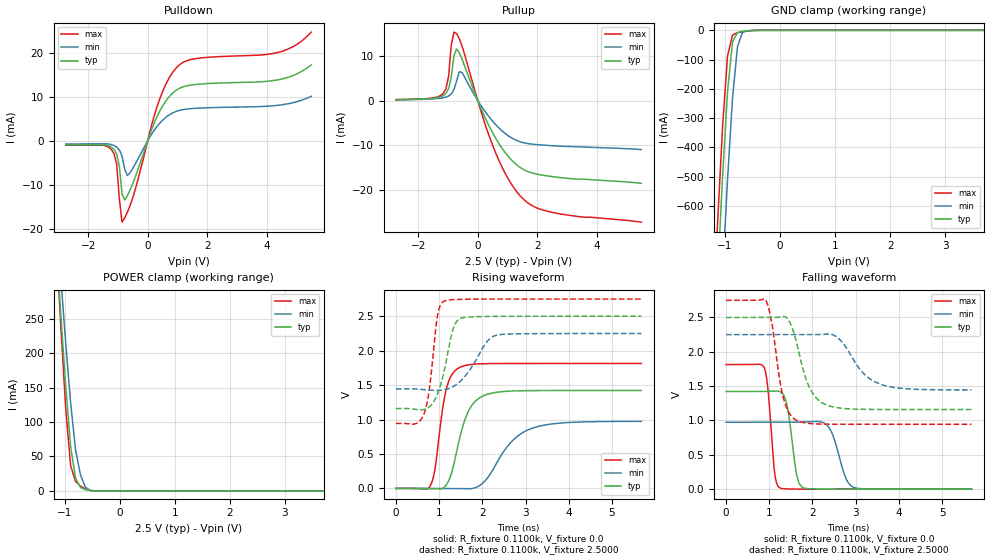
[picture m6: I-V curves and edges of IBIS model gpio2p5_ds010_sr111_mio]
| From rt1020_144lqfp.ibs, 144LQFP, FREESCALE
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[Model] gpio2p5_ds010_sr111_mio
|   Model gpio2p5_ds010_sr111_mio
| This model was characterised for following simulation conditions:
| External (pad) voltage:
|   - Typ: 2.5V,   - Min: 2.25V,   - Max: 2.75V
| Library cells for typ/min/max conditions are connected as defined below:
|  pad - External Pad
|  ipp_do - Core Input
|  ipp_obe - Output Buffer Enable
|  esd_boost - ovdd
|  ipp_dse0 - vssi
|  ipp_dse1 - vddi
|  ipp_dse2 - vssi
|  ipp_fsel0 - vddi
|  ipp_fsel1 - vddi
|  ipp_ina - ipp_ina
|  ipp_ind - ipp_ind
|  ipp_pwr_stable - vddi
|  ipp_sre - vddi
|  ovdd - ovdd
|  ovss - ovss
|  vddi - vddi
|  vssi - vssi
| All other pins connected to ground
Model_type I/O
Polarity   Non-Inverting
Enable   Active-High
Vinl =   0.7500V
Vinh =   1.7500V
Vmeas =  1.2500V
Cref =   0.0F
Rref =   0.1100k
Vref =   1.2500V
C_comp   1.2356pF   1.1994pF   1.2834pF
|C_comp_pullup   0.6222pF   0.6389pF   0.6073pF
|C_comp_pulldown   0.5474pF   0.5788pF   0.5258pF
[Model Spec]
| variable   typ   min   max
Vinh   1.7500V   1.5750V   1.9250V
Vinl   0.7500V   0.6750V   0.8250V
S_overshoot_high   2.5000V   2.2500V   2.7500V
S_overshoot_low   0.0V   0.0V   0.0V
Vmeas   1.2500V   1.1250V   1.3750V
Vref   1.2500V   1.1250V   1.3750V
Cref   0.0F   0.0F   0.0F
Rref   0.1100k   0.1100k   0.1100k
[Temperature Range]   25.0000   0.1050k   -20.0000
[Voltage Range]   2.5000V   2.2500V   2.7500V
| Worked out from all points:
|   slope of the pulldown table from 0 to 0.375 V, typ, clamps not added: 59.2 ohm
|   slope of the pullup table from 0 to 0.375 V, typ, clamps not added: 66.8 ohm
|   GND clamp passes 1 mA (typ) near -0.54 V on its own axis
|   POWER clamp passes 1 mA (typ) near -0.57 V on its own axis
|   rising waveform, R_fixture 0.1100k, V_fixture 0.0: 20-80 % time 377ps typ, 690ps min, 246ps max; typ from 0 V to 1.42 V
|   rising waveform, R_fixture 0.1100k, V_fixture 2.5000: 20-80 % time 292ps typ, 492ps min, 194ps max; typ from 1.16 V to 2.5 V
|   falling waveform, R_fixture 0.1100k, V_fixture 0.0: 20-80 % time 177ps typ, 276ps min, 133ps max; typ from 1.42 V to 0 V
|   falling waveform, R_fixture 0.1100k, V_fixture 2.5000: 20-80 % time 384ps typ, 583ps min, 269ps max; typ from 2.5 V to 1.16 V
[Pulldown]
|Voltage   I(typ)   I(min)   I(max)
-2.75V    -867uA     -694uA     -970uA
-1.22V    -1.39mA    -820uA     -1.909mA
-1.04V    -2.968mA   -1.376mA   -5.261mA
-950mV    -5.74mA    -2.023mA   -13.11mA
-860mV    -11.97mA   -3.453mA   -18.4mA
-770mV    -13.39mA   -6.394mA   -17.42mA
-680mV    -12.38mA   -7.845mA   -16.13mA
400mV     6.671mA    3.97mA     9.391mA
1.03V     11.78mA    6.858mA    17.01mA
1.66V     12.83mA    7.418mA    18.71mA
4.36V     13.84mA    8.07mA     20.03mA
5.5V      17.23mA    10.11mA    24.67mA
[Pullup]
|Voltage   I(typ)   I(min)   I(max)
-2.75V    180uA      160uA      200uA
-1.16V    1.087mA    609uA      1.595mA
-980mV    2.638mA    1.014mA    5.407mA
-890mV    5.313mA    1.485mA    12.39mA
-800mV    10.05mA    2.436mA    15.32mA
-710mV    11.53mA    4.364mA    14.98mA
-620mV    10.67mA    6.425mA    13.85mA
-530mV    9.303mA    6.294mA    12.25mA
550mV     -7.823mA   -5.015mA   -10.85mA
1.45V     -15.1mA    -9.298mA   -21.52mA
2.53V     -17.06mA   -10.13mA   -25.08mA
5.5V      -18.54mA   -10.99mA   -27.24mA
[GND_clamp]
|Voltage   I(typ)   I(min)   I(max)
-2.75V    -7.488A    -7.708A    -7.379A
-1.22V    -1.193A    -1.537A    -1.012A
-1.13V    -835.6mA   -1.18A     -654.7mA
-1.04V    -497.8mA   -833mA     -328mA
-950mV    -208.9mA   -508.7mA   -87.54mA
-860mV    -39.89mA   -232.5mA   -15.89mA
-770mV    -7.264mA   -56.44mA   -8.363mA
-680mV    -3.422mA   -7.048mA   -4.851mA
-590mV    -1.552mA   -1.455mA   -2.251mA
-500mV    -482.7uA   -438.2uA   -698.4uA
5.5V      0A         0A         0A
[POWER_clamp]
|Voltage   I(typ)   I(min)   I(max)
-2.75V    2.386A     2.288A     2.687A
-1.16V    368.2mA    410.8mA    372.9mA
-1.07V    258.5mA    311.8mA    242.5mA
-980mV    153.1mA    216.2mA    121.1mA
-890mV    64.5mA     128mA      36.56mA
-800mV    18.16mA    59.6mA     13.82mA
-710mV    5.012mA    22.76mA    6.935mA
-620mV    1.706mA    5.315mA    2.959mA
-530mV    383.1uA    636.8uA    795.1uA
-440mV    42.36uA    66.97uA    84.45uA
5.5V      0A         0A         0A
[Ramp]
| variable   typ   min   max
dV/dt_r  0.8532/0.3773n   0.5844/0.6905n   1.0887/0.2460n
dV/dt_f  0.8044/0.3836n   0.4831/0.5828n   1.0834/0.2693n
R_load = 0.1100k
[Rising Waveform]
R_fixture= 0.1100k
V_fixture= 0.0
V_fixture_min= 0.0
V_fixture_max= 0.0
|time   V(typ)   V(min)   V(max)
0s        1.854nV    7.26nV     5.849nV
795.6ps   -3.358mV   216.2uV    37.43mV
904.6ps   -6.093mV   -847nV     283.8mV
1.169ns   54.48mV    -1.241mV   1.451V
1.463ns   697.6mV    -4.061mV   1.753V
1.748ns   1.198V     -2.93mV    1.801V
2.182ns   1.379V     207.1mV    1.813V
2.627ns   1.413V     645.6mV    1.814V
3.114ns   1.42V      865mV      1.814V
5.68ns    1.422V     974mV      1.814V
[Rising Waveform]
R_fixture= 0.1100k
V_fixture= 2.5000
V_fixture_min= 2.2500
V_fixture_max= 2.7500
|time   V(typ)   V(min)   V(max)
0s        1.159V     1.444V     944.2mV
466.5ps   1.145V     1.445V     941.3mV
651.4ps   1.146V     1.434V     1.084V
771.8ps   1.184V     1.428V     1.432V
963.7ps   1.375V     1.423V     2.514V
1.111ns   1.689V     1.432V     2.719V
1.334ns   2.335V     1.482V     2.742V
1.523ns   2.475V     1.577V     2.747V
2.314ns   2.499V     2.223V     2.75V
5.68ns    2.5V       2.25V      2.75V
[Falling Waveform]
R_fixture= 0.1100k
V_fixture= 0.0
V_fixture_min= 0.0
V_fixture_max= 0.0
|time   V(typ)   V(min)   V(max)
0s        1.422V     974.5mV    1.814V
880.2ps   1.423V     974.2mV    1.772V
978.3ps   1.425V     974.2mV    1.402V
1.12ns    1.429V     974.2mV    263.2mV
1.241ns   1.421V     974.3mV    20.77mV
1.395ns   1.266V     974.5mV    3.972mV
1.789ns   20.3mV     978.6mV    664.2uV
2.372ns   926.6uV    907mV      177.2uV
2.939ns   235.6uV    29.99mV    81.13uV
5.68ns    11.64uV    33.62uV    -1.492uV
[Falling Waveform]
R_fixture= 0.1100k
V_fixture= 2.5000
V_fixture_min= 2.2500
V_fixture_max= 2.7500
|time   V(typ)   V(min)   V(max)
0s        2.5V       2.25V      2.75V
924.5ps   2.5V       2.25V      2.745V
1.061ns   2.499V     2.25V      2.414V
1.33ns    2.514V     2.25V      1.322V
1.487ns   2.415V     2.25V      1.084V
1.653ns   2.081V     2.25V      996.4mV
1.942ns   1.465V     2.25V      955.9mV
2.327ns   1.226V     2.258V     946.2mV
3.546ns   1.16V      1.535V     944.4mV
5.68ns    1.159V     1.445V     944.3mV
